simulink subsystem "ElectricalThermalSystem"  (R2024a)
settings: Solver=VariableStepAuto  StartTime=0.0  StopTime=10.0  RelTol=1e-3
undefined symbols (not defined in the file): EnvAirTemp, PlantThrEstCmpPwr, PlntThrAirBpt, PlntThrAirCond, PlntThrAirCp, PlntThrAirCpBpt, PlntThrAirPrand, PlntThrAirRho, PlntThrAirVisc, PlntThrBattDCFlwRatio, PlntThrBattJacLen, PlntThrChArea, PlntThrChDia, PlntThrCoolCond, PlntThrCoolCp, PlntThrCoolCpBpt, PlntThrCoolPrand, PlntThrCoolRho, PlntThrCoolVisc, PlntThrDCJacLen, PlntThrEMJacLen, PlntThrEstCOPLut, PlntThrEstDTLut, PlntThrHeaterMaxPwr, PlntThrPmpDisp, PlntThrPmpHeadP, PlntThrPmpMaxSpd, PlntThrPmpMechEff, PlntThrPmpVolEff, PlntThrRadAirArea, PlntThrRadAirDh, PlntThrRadFanAreaFlw, PlntThrRadFlwCoef, PlntThrRadGapHeight, PlntThrRadLength, PlntThrRadNTubes, PlntThrRadTubeDh, PlntThrRadTubeHeight, PlntThrRadWidth
libraries: autolibutils x45
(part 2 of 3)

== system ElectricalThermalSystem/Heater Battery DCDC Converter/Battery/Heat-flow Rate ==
  HTC : Inport
  JacHtArea : Inport  Port=2
  BattTemp : Inport  Port=3
  CoolBlkTemp : Inport  Port=4
  Product2 : Product  Inputs=3
  Subtract1 : Sum  Inputs=+-
  Qbatt : Outport
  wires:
  BattTemp/1 -> Subtract1/1
  Product2/1 -> Qbatt/1
  CoolBlkTemp/1 -> Subtract1/2
  JacHtArea/1 -> Product2/2
  Subtract1/1 -> Product2/3
  HTC/1 -> Product2/1

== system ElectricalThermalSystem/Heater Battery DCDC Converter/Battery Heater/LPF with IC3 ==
  u : Inport
  Cont LPF IC : autolibutils/Cont LPF IC  wc=wc  aMode=1  dataType=off
  Initial Condition : Constant  Value=InitCond  SampleTime=-1
  y : Outport
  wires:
  Cont LPF IC/1 -> y/1
  u/1 -> Cont LPF IC/1
  Initial Condition/1 -> Cont LPF IC/2

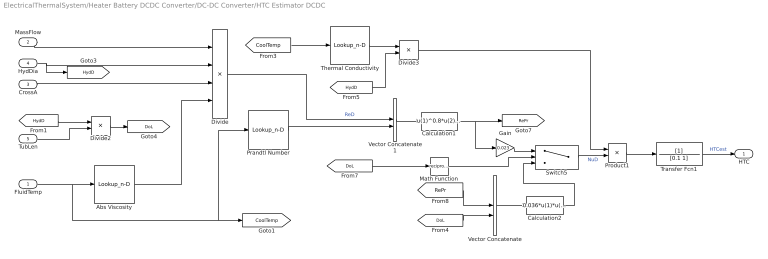
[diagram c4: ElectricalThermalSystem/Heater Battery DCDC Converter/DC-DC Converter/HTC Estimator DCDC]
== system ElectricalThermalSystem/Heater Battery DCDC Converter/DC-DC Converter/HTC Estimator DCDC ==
  FluidTemp : Inport
  MassFlow : Inport  Port=2
  CrossA : Inport  Port=3  OutMin=eps
  HydDia : Inport  Port=4
  TubLen : Inport  Port=5
  Abs Viscosity : Lookup_n-D  NumberOfTableDimensions=1  BreakpointsForDimension1=PlntThrCoolCpBpt  Table=PlntThrCoolVisc  ExtrapMethod=Clip  UseLastTableValue=on  InternalRulePriority=Speed  RndMeth=Simplest
  Calculation1 : Fcn  Expr=u(1)^0.8*u(2)^0.33
  Calculation2 : Fcn  Expr=0.036*u(1)*u(2)^0.055
  Divide : Product  Inputs=**//
  Divide2 : Product  Inputs=*/
  Divide3 : Product  Inputs=*/
  Gain : Gain  Gain=0.023
  Math Function : Math  Operator=reciprocal
  Prandtl Number : Lookup_n-D  NumberOfTableDimensions=1  BreakpointsForDimension1=PlntThrCoolCpBpt  Table=PlntThrCoolPrand  ExtrapMethod=Clip  UseLastTableValue=on  InternalRulePriority=Speed  RndMeth=Simplest
  Product1 : Product
  Switch5 : Switch  Threshold=400
  Thermal Conductivity : Lookup_n-D  NumberOfTableDimensions=1  BreakpointsForDimension1=PlntThrCoolCpBpt  Table=PlntThrCoolCond  ExtrapMethod=Clip  UseLastTableValue=on  InternalRulePriority=Speed  RndMeth=Simplest
  Transfer Fcn1 : TransferFcn  Denominator=[0.1 1]
  Vector Concatenate : Concatenate
  Vector Concatenate1 : Concatenate
  HTC : Outport
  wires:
  Product1/1 -> Transfer Fcn1/1
  Switch5/1 -> Product1/2  "NuD"
  Calculation2/1 -> Switch5/3
  Vector Concatenate/1 -> Calculation2/1
  [DoL] -> Vector Concatenate/2
  [RePr] -> Vector Concatenate/1
  Calculation1/1 -> Gain/1, [RePr]
  Gain/1 -> Switch5/1
  Divide3/1 -> Product1/1
  [HydD] -> Divide3/2
  Thermal Conductivity/1 -> Divide3/1
  Math Function/1 -> Switch5/2
  [DoL] -> Math Function/1
  Vector Concatenate1/1 -> Calculation1/1
  Prandtl Number/1 -> Vector Concatenate1/2
  Divide/1 -> Vector Concatenate1/1  "ReD"
  Abs Viscosity/1 -> Divide/4
  Divide2/1 -> [DoL]
  TubLen/1 -> Divide2/2
  [HydD] -> Divide2/1
  CrossA/1 -> Divide/3
  HydDia/1 -> Divide/2, [HydD]
  MassFlow/1 -> Divide/1
  [CoolTemp] -> Thermal Conductivity/1
  FluidTemp/1 -> Abs Viscosity/1, [CoolTemp], Prandtl Number/1
  Transfer Fcn1/1 -> HTC/1  "HTCest"

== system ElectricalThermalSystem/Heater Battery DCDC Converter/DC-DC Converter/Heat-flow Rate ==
  HTC : Inport
  PwrETemp : Inport  Port=2
  JacArea : Inport  Port=3
  CoolBlkTemp : Inport  Port=4
  Product1 : Product  Inputs=3
  Subtract : Sum  Inputs=+-
  Qpwre : Outport
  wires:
  HTC/1 -> Product1/1
  Product1/1 -> Qpwre/1
  CoolBlkTemp/1 -> Subtract/2
  PwrETemp/1 -> Subtract/1
  Subtract/1 -> Product1/3
  JacArea/1 -> Product1/2

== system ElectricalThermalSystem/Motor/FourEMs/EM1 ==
  CoolTempIn : Inport
  CoolMFlow : Inport  Port=2
  EMTemp : Inport  Port=3
  Constant : Constant  Value=JacHtArea  SampleTime=-1
  Constant1 : Constant  Value=JacDia
  Constant2 : Constant  Value=JacArea
  Constant3 : Constant  Value=JacLen
  HTC Estimator EM : Subsystem
  Temperature and Heat Flow : Subsystem
  Qem : Outport
  CoolTempOut : Outport  Port=2
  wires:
  Constant/1 -> Temperature and Heat Flow/5(JacArea)
  CoolTempIn/1 -> Temperature and Heat Flow/2(CoolTempIn)
  Temperature and Heat Flow/3(CoolTempOut) -> CoolTempOut/1
  Temperature and Heat Flow/2(Qem) -> Qem/1
  Constant2/1 -> HTC Estimator EM/3(CrossA)
  [BulkCoolTemp] -> HTC Estimator EM/1(FluidTemp)
  Constant3/1 -> HTC Estimator EM/5(TubLen)
  EMTemp/1 -> Temperature and Heat Flow/3(EMTemp)
  [CoolMFlw] -> Temperature and Heat Flow/4(CoolMflw)
  CoolMFlow/1 -> [CoolMFlw], HTC Estimator EM/2(MassFlow)
  HTC Estimator EM/1(HTC) -> Temperature and Heat Flow/1(HTC)
  Temperature and Heat Flow/1(BulkCoolTemp) -> [BulkCoolTemp]
  Constant1/1 -> HTC Estimator EM/4(HydDia)

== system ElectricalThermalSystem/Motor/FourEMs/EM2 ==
  CoolTempIn : Inport
  CoolMFlow : Inport  Port=2
  EMTemp : Inport  Port=3
  Constant : Constant  Value=JacHtArea  SampleTime=-1
  Constant1 : Constant  Value=JacDia
  Constant2 : Constant  Value=JacArea
  Constant3 : Constant  Value=JacLen
  HTC Estimator EM : Subsystem
  Temperature and Heat Flow : Subsystem
  Qem : Outport
  CoolTempOut : Outport  Port=2
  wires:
  Constant/1 -> Temperature and Heat Flow/5(JacArea)
  CoolTempIn/1 -> Temperature and Heat Flow/2(CoolTempIn)
  Temperature and Heat Flow/3(CoolTempOut) -> CoolTempOut/1
  Temperature and Heat Flow/2(Qem) -> Qem/1
  Constant2/1 -> HTC Estimator EM/3(CrossA)
  [BulkCoolTemp] -> HTC Estimator EM/1(FluidTemp)
  Constant3/1 -> HTC Estimator EM/5(TubLen)
  EMTemp/1 -> Temperature and Heat Flow/3(EMTemp)
  [CoolMFlw] -> Temperature and Heat Flow/4(CoolMflw)
  CoolMFlow/1 -> [CoolMFlw], HTC Estimator EM/2(MassFlow)
  HTC Estimator EM/1(HTC) -> Temperature and Heat Flow/1(HTC)
  Temperature and Heat Flow/1(BulkCoolTemp) -> [BulkCoolTemp]
  Constant1/1 -> HTC Estimator EM/4(HydDia)

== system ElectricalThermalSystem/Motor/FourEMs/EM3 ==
  CoolTempIn : Inport
  CoolMFlow : Inport  Port=2
  EMTemp : Inport  Port=3
  Constant : Constant  Value=JacHtArea  SampleTime=-1
  Constant1 : Constant  Value=JacDia
  Constant2 : Constant  Value=JacArea
  Constant3 : Constant  Value=JacLen
  HTC Estimator EM : Subsystem
  Temperature and Heat Flow : Subsystem
  Qem : Outport
  CoolTempOut : Outport  Port=2
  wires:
  Constant/1 -> Temperature and Heat Flow/5(JacArea)
  CoolTempIn/1 -> Temperature and Heat Flow/2(CoolTempIn)
  Temperature and Heat Flow/3(CoolTempOut) -> CoolTempOut/1
  Temperature and Heat Flow/2(Qem) -> Qem/1
  Constant2/1 -> HTC Estimator EM/3(CrossA)
  [BulkCoolTemp] -> HTC Estimator EM/1(FluidTemp)
  Constant3/1 -> HTC Estimator EM/5(TubLen)
  EMTemp/1 -> Temperature and Heat Flow/3(EMTemp)
  [CoolMFlw] -> Temperature and Heat Flow/4(CoolMflw)
  CoolMFlow/1 -> [CoolMFlw], HTC Estimator EM/2(MassFlow)
  HTC Estimator EM/1(HTC) -> Temperature and Heat Flow/1(HTC)
  Temperature and Heat Flow/1(BulkCoolTemp) -> [BulkCoolTemp]
  Constant1/1 -> HTC Estimator EM/4(HydDia)

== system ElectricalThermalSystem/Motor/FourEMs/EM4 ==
  CoolTempIn : Inport
  CoolMFlow : Inport  Port=2
  EMTemp : Inport  Port=3
  Constant : Constant  Value=JacHtArea  SampleTime=-1
  Constant1 : Constant  Value=JacDia
  Constant2 : Constant  Value=JacArea
  Constant3 : Constant  Value=JacLen
  HTC Estimator EM : Subsystem
  Temperature and Heat Flow : Subsystem
  Qem : Outport
  CoolTempOut : Outport  Port=2
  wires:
  Constant/1 -> Temperature and Heat Flow/5(JacArea)
  CoolTempIn/1 -> Temperature and Heat Flow/2(CoolTempIn)
  Temperature and Heat Flow/3(CoolTempOut) -> CoolTempOut/1
  Temperature and Heat Flow/2(Qem) -> Qem/1
  Constant2/1 -> HTC Estimator EM/3(CrossA)
  [BulkCoolTemp] -> HTC Estimator EM/1(FluidTemp)
  Constant3/1 -> HTC Estimator EM/5(TubLen)
  EMTemp/1 -> Temperature and Heat Flow/3(EMTemp)
  [CoolMFlw] -> Temperature and Heat Flow/4(CoolMflw)
  CoolMFlow/1 -> [CoolMFlw], HTC Estimator EM/2(MassFlow)
  HTC Estimator EM/1(HTC) -> Temperature and Heat Flow/1(HTC)
  Temperature and Heat Flow/1(BulkCoolTemp) -> [BulkCoolTemp]
  Constant1/1 -> HTC Estimator EM/4(HydDia)

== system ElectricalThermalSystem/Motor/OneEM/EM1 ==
  MassFlow : Inport
  CoolTempIn : Inport  Port=2
  EMTemp : Inport  Port=3
  Constant : Constant  Value=JacHtArea  SampleTime=-1
  Constant1 : Constant  Value=JacDia
  Constant2 : Constant  Value=JacArea
  Constant3 : Constant  Value=JacLen
  HTC Estimator EM : Subsystem
  Temperature and Heat Flow : Subsystem
  Qem : Outport
  CoolTempOut : Outport  Port=2
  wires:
  Constant/1 -> Temperature and Heat Flow/5(JacArea)
  CoolTempIn/1 -> Temperature and Heat Flow/2(CoolTempIn)
  Temperature and Heat Flow/3(CoolTempOut) -> CoolTempOut/1
  Temperature and Heat Flow/2(Qem) -> Qem/1
  Constant2/1 -> HTC Estimator EM/3(CrossA)
  [BulkCoolTemp] -> HTC Estimator EM/1(FluidTemp)
  Constant3/1 -> HTC Estimator EM/5(TubLen)
  EMTemp/1 -> Temperature and Heat Flow/3(EMTemp)
  [CoolMFlw] -> Temperature and Heat Flow/4(CoolMflw)
  MassFlow/1 -> [CoolMFlw], HTC Estimator EM/2(MassFlow)
  HTC Estimator EM/1(HTC) -> Temperature and Heat Flow/1(HTC)
  Temperature and Heat Flow/1(BulkCoolTemp) -> [BulkCoolTemp]
  Constant1/1 -> HTC Estimator EM/4(HydDia)

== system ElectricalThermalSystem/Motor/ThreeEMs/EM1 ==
  CoolTempIn : Inport
  CoolMFlow : Inport  Port=2
  EMTemp : Inport  Port=3
  Constant : Constant  Value=JacHtArea  SampleTime=-1
  Constant1 : Constant  Value=JacDia
  Constant2 : Constant  Value=JacArea
  Constant3 : Constant  Value=JacLen
  HTC Estimator EM : Subsystem
  Temperature and Heat Flow : Subsystem
  Qem : Outport
  CoolTempOut : Outport  Port=2
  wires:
  Constant/1 -> Temperature and Heat Flow/5(JacArea)
  CoolTempIn/1 -> Temperature and Heat Flow/2(CoolTempIn)
  Temperature and Heat Flow/3(CoolTempOut) -> CoolTempOut/1
  Temperature and Heat Flow/2(Qem) -> Qem/1
  Constant2/1 -> HTC Estimator EM/3(CrossA)
  [BulkCoolTemp] -> HTC Estimator EM/1(FluidTemp)
  Constant3/1 -> HTC Estimator EM/5(TubLen)
  EMTemp/1 -> Temperature and Heat Flow/3(EMTemp)
  [CoolMFlw] -> Temperature and Heat Flow/4(CoolMflw)
  CoolMFlow/1 -> [CoolMFlw], HTC Estimator EM/2(MassFlow)
  HTC Estimator EM/1(HTC) -> Temperature and Heat Flow/1(HTC)
  Temperature and Heat Flow/1(BulkCoolTemp) -> [BulkCoolTemp]
  Constant1/1 -> HTC Estimator EM/4(HydDia)

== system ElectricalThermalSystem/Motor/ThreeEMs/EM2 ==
  CoolTempIn : Inport
  CoolMFlow : Inport  Port=2
  EMTemp : Inport  Port=3
  Constant : Constant  Value=JacHtArea  SampleTime=-1
  Constant1 : Constant  Value=JacDia
  Constant2 : Constant  Value=JacArea
  Constant3 : Constant  Value=JacLen
  HTC Estimator EM : Subsystem
  Temperature and Heat Flow : Subsystem
  Qem : Outport
  CoolTempOut : Outport  Port=2
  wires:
  Constant/1 -> Temperature and Heat Flow/5(JacArea)
  CoolTempIn/1 -> Temperature and Heat Flow/2(CoolTempIn)
  Temperature and Heat Flow/3(CoolTempOut) -> CoolTempOut/1
  Temperature and Heat Flow/2(Qem) -> Qem/1
  Constant2/1 -> HTC Estimator EM/3(CrossA)
  [BulkCoolTemp] -> HTC Estimator EM/1(FluidTemp)
  Constant3/1 -> HTC Estimator EM/5(TubLen)
  EMTemp/1 -> Temperature and Heat Flow/3(EMTemp)
  [CoolMFlw] -> Temperature and Heat Flow/4(CoolMflw)
  CoolMFlow/1 -> [CoolMFlw], HTC Estimator EM/2(MassFlow)
  HTC Estimator EM/1(HTC) -> Temperature and Heat Flow/1(HTC)
  Temperature and Heat Flow/1(BulkCoolTemp) -> [BulkCoolTemp]
  Constant1/1 -> HTC Estimator EM/4(HydDia)

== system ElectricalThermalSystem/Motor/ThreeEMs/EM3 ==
  CoolTempIn : Inport
  CoolMFlow : Inport  Port=2
  EMTemp : Inport  Port=3
  Constant : Constant  Value=JacHtArea  SampleTime=-1
  Constant1 : Constant  Value=JacDia
  Constant2 : Constant  Value=JacArea
  Constant3 : Constant  Value=JacLen
  HTC Estimator EM : Subsystem
  Temperature and Heat Flow : Subsystem
  Qem : Outport
  CoolTempOut : Outport  Port=2
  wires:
  Constant/1 -> Temperature and Heat Flow/5(JacArea)
  CoolTempIn/1 -> Temperature and Heat Flow/2(CoolTempIn)
  Temperature and Heat Flow/3(CoolTempOut) -> CoolTempOut/1
  Temperature and Heat Flow/2(Qem) -> Qem/1
  Constant2/1 -> HTC Estimator EM/3(CrossA)
  [BulkCoolTemp] -> HTC Estimator EM/1(FluidTemp)
  Constant3/1 -> HTC Estimator EM/5(TubLen)
  EMTemp/1 -> Temperature and Heat Flow/3(EMTemp)
  [CoolMFlw] -> Temperature and Heat Flow/4(CoolMflw)
  CoolMFlow/1 -> [CoolMFlw], HTC Estimator EM/2(MassFlow)
  HTC Estimator EM/1(HTC) -> Temperature and Heat Flow/1(HTC)
  Temperature and Heat Flow/1(BulkCoolTemp) -> [BulkCoolTemp]
  Constant1/1 -> HTC Estimator EM/4(HydDia)

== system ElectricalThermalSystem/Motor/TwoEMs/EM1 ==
  CoolTempIn : Inport
  CoolMFlow : Inport  Port=2
  EMTemp : Inport  Port=3
  Constant : Constant  Value=JacHtArea  SampleTime=-1
  Constant1 : Constant  Value=JacDia
  Constant2 : Constant  Value=JacArea
  Constant3 : Constant  Value=JacLen
  HTC Estimator EM : Subsystem
  Temperature and Heat Flow : Subsystem
  Qem : Outport
  CoolTempOut : Outport  Port=2
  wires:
  Constant/1 -> Temperature and Heat Flow/5(JacArea)
  CoolTempIn/1 -> Temperature and Heat Flow/2(CoolTempIn)
  Temperature and Heat Flow/3(CoolTempOut) -> CoolTempOut/1
  Temperature and Heat Flow/2(Qem) -> Qem/1
  Constant2/1 -> HTC Estimator EM/3(CrossA)
  [BulkCoolTemp] -> HTC Estimator EM/1(FluidTemp)
  Constant3/1 -> HTC Estimator EM/5(TubLen)
  EMTemp/1 -> Temperature and Heat Flow/3(EMTemp)
  [CoolMFlw] -> Temperature and Heat Flow/4(CoolMflw)
  CoolMFlow/1 -> [CoolMFlw], HTC Estimator EM/2(MassFlow)
  HTC Estimator EM/1(HTC) -> Temperature and Heat Flow/1(HTC)
  Temperature and Heat Flow/1(BulkCoolTemp) -> [BulkCoolTemp]
  Constant1/1 -> HTC Estimator EM/4(HydDia)

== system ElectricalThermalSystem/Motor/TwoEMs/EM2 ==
  CoolTempIn : Inport
  CoolMFlow : Inport  Port=2
  EMTemp : Inport  Port=3
  Constant : Constant  Value=JacHtArea  SampleTime=-1
  Constant1 : Constant  Value=JacDia
  Constant2 : Constant  Value=JacArea
  Constant3 : Constant  Value=JacLen
  HTC Estimator EM : Subsystem
  Temperature and Heat Flow : Subsystem
  Qem : Outport
  CoolTempOut : Outport  Port=2
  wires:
  Constant/1 -> Temperature and Heat Flow/5(JacArea)
  CoolTempIn/1 -> Temperature and Heat Flow/2(CoolTempIn)
  Temperature and Heat Flow/3(CoolTempOut) -> CoolTempOut/1
  Temperature and Heat Flow/2(Qem) -> Qem/1
  Constant2/1 -> HTC Estimator EM/3(CrossA)
  [BulkCoolTemp] -> HTC Estimator EM/1(FluidTemp)
  Constant3/1 -> HTC Estimator EM/5(TubLen)
  EMTemp/1 -> Temperature and Heat Flow/3(EMTemp)
  [CoolMFlw] -> Temperature and Heat Flow/4(CoolMflw)
  CoolMFlow/1 -> [CoolMFlw], HTC Estimator EM/2(MassFlow)
  HTC Estimator EM/1(HTC) -> Temperature and Heat Flow/1(HTC)
  Temperature and Heat Flow/1(BulkCoolTemp) -> [BulkCoolTemp]
  Constant1/1 -> HTC Estimator EM/4(HydDia)

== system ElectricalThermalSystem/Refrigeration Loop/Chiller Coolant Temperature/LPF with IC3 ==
  u : Inport
  Cont LPF IC : autolibutils/Cont LPF IC  wc=wc  aMode=1  dataType=off
  Initial Condition : Constant  Value=InitCond  SampleTime=-1
  y : Outport
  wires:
  Cont LPF IC/1 -> y/1
  u/1 -> Cont LPF IC/1
  Initial Condition/1 -> Cont LPF IC/2

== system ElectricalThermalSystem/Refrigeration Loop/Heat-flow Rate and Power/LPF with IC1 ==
  u : Inport
  Cont LPF IC : autolibutils/Cont LPF IC  wc=wc  aMode=1  dataType=off
  Initial Condition : Constant  Value=InitCond  SampleTime=-1
  y : Outport
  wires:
  Cont LPF IC/1 -> y/1
  u/1 -> Cont LPF IC/1
  Initial Condition/1 -> Cont LPF IC/2

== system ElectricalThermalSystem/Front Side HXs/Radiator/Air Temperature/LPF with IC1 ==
  u : Inport
  Cont LPF IC : autolibutils/Cont LPF IC  wc=wc  aMode=1  dataType=off
  Initial Condition : Constant  Value=InitCond  SampleTime=-1
  y : Outport
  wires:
  Cont LPF IC/1 -> y/1
  u/1 -> Cont LPF IC/1
  Initial Condition/1 -> Cont LPF IC/2

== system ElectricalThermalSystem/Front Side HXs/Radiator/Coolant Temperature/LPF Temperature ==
  u : Inport
  Cont LPF IC : autolibutils/Cont LPF IC  wc=wc  aMode=1  dataType=off
  Initial Condition : Constant  Value=InitCond  SampleTime=-1
  y : Outport
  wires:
  Cont LPF IC/1 -> y/1
  u/1 -> Cont LPF IC/1
  Initial Condition/1 -> Cont LPF IC/2

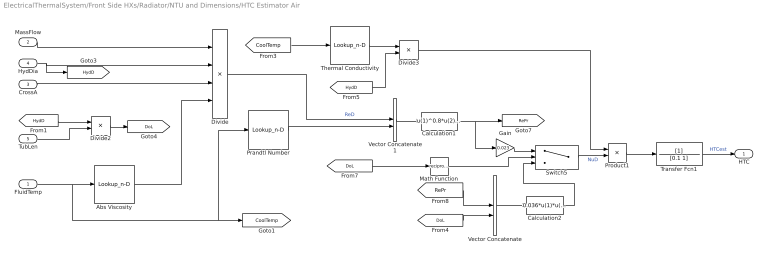
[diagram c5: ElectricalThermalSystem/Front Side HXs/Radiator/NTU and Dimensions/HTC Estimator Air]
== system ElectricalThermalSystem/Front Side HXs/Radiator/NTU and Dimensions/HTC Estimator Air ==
  FluidTemp : Inport
  MassFlow : Inport  Port=2
  CrossA : Inport  Port=3  OutMin=eps
  HydDia : Inport  Port=4
  TubLen : Inport  Port=5
  Abs Viscosity : Lookup_n-D  NumberOfTableDimensions=1  BreakpointsForDimension1=PlntThrAirCpBpt  Table=PlntThrAirVisc  ExtrapMethod=Clip  UseLastTableValue=on  InternalRulePriority=Speed  RndMeth=Simplest
  Calculation1 : Fcn  Expr=u(1)^0.8*u(2)^0.33
  Calculation2 : Fcn  Expr=0.036*u(1)*u(2)^0.055
  Divide : Product  Inputs=**//
  Divide2 : Product  Inputs=*/
  Divide3 : Product  Inputs=*/
  Gain : Gain  Gain=0.023
  Math Function : Math  Operator=reciprocal
  Prandtl Number : Lookup_n-D  NumberOfTableDimensions=1  BreakpointsForDimension1=PlntThrAirCpBpt  Table=PlntThrAirPrand  ExtrapMethod=Clip  UseLastTableValue=on  InternalRulePriority=Speed  RndMeth=Simplest
  Product1 : Product
  Switch5 : Switch  Threshold=400
  Thermal Conductivity : Lookup_n-D  NumberOfTableDimensions=1  BreakpointsForDimension1=PlntThrAirCpBpt  Table=PlntThrAirCond  ExtrapMethod=Clip  UseLastTableValue=on  InternalRulePriority=Speed  RndMeth=Simplest
  Transfer Fcn1 : TransferFcn  Denominator=[0.1 1]
  Vector Concatenate : Concatenate
  Vector Concatenate1 : Concatenate
  HTC : Outport
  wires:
  MassFlow/1 -> Divide/1
  Product1/1 -> Transfer Fcn1/1
  Switch5/1 -> Product1/2  "NuD"
  Calculation2/1 -> Switch5/3
  Vector Concatenate/1 -> Calculation2/1
  [DoL] -> Vector Concatenate/2
  [RePr] -> Vector Concatenate/1
  Calculation1/1 -> Gain/1, [RePr]
  Gain/1 -> Switch5/1
  Divide3/1 -> Product1/1
  [HydD] -> Divide3/2
  Thermal Conductivity/1 -> Divide3/1
  Math Function/1 -> Switch5/2
  [DoL] -> Math Function/1
  Vector Concatenate1/1 -> Calculation1/1
  Prandtl Number/1 -> Vector Concatenate1/2
  Divide/1 -> Vector Concatenate1/1  "ReD"
  Abs Viscosity/1 -> Divide/4
  Divide2/1 -> [DoL]
  TubLen/1 -> Divide2/2
  [HydD] -> Divide2/1
  CrossA/1 -> Divide/3
  HydDia/1 -> Divide/2, [HydD]
  [CoolTemp] -> Thermal Conductivity/1
  FluidTemp/1 -> Abs Viscosity/1, [CoolTemp], Prandtl Number/1
  Transfer Fcn1/1 -> HTC/1  "HTCest"

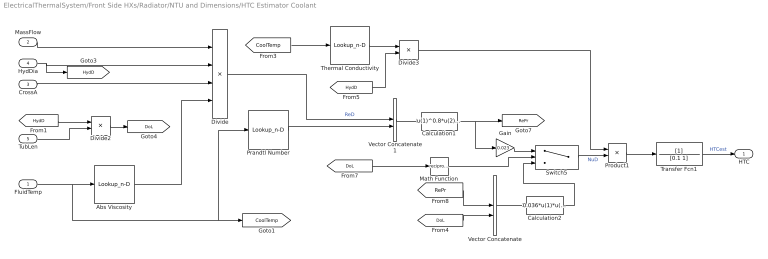
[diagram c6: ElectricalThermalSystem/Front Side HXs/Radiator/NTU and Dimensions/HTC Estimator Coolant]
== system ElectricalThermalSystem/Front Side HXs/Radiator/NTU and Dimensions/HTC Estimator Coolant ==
  FluidTemp : Inport
  MassFlow : Inport  Port=2
  CrossA : Inport  Port=3  OutMin=eps
  HydDia : Inport  Port=4
  TubLen : Inport  Port=5
  Abs Viscosity : Lookup_n-D  NumberOfTableDimensions=1  BreakpointsForDimension1=PlntThrCoolCpBpt  Table=PlntThrCoolVisc  ExtrapMethod=Clip  UseLastTableValue=on  InternalRulePriority=Speed  RndMeth=Simplest
  Calculation1 : Fcn  Expr=u(1)^0.8*u(2)^0.33
  Calculation2 : Fcn  Expr=0.036*u(1)*u(2)^0.055
  Divide : Product  Inputs=**//
  Divide2 : Product  Inputs=*/
  Divide3 : Product  Inputs=*/
  Gain : Gain  Gain=0.023
  Math Function : Math  Operator=reciprocal
  Prandtl Number : Lookup_n-D  NumberOfTableDimensions=1  BreakpointsForDimension1=PlntThrCoolCpBpt  Table=PlntThrCoolPrand  ExtrapMethod=Clip  UseLastTableValue=on  InternalRulePriority=Speed  RndMeth=Simplest
  Product1 : Product
  Switch5 : Switch  Threshold=400
  Thermal Conductivity : Lookup_n-D  NumberOfTableDimensions=1  BreakpointsForDimension1=PlntThrCoolCpBpt  Table=PlntThrCoolCond  ExtrapMethod=Clip  UseLastTableValue=on  InternalRulePriority=Speed  RndMeth=Simplest
  Transfer Fcn1 : TransferFcn  Denominator=[0.1 1]
  Vector Concatenate : Concatenate
  Vector Concatenate1 : Concatenate
  HTC : Outport
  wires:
  MassFlow/1 -> Divide/1
  Product1/1 -> Transfer Fcn1/1
  Switch5/1 -> Product1/2  "NuD"
  Calculation2/1 -> Switch5/3
  Vector Concatenate/1 -> Calculation2/1
  [DoL] -> Vector Concatenate/2
  [RePr] -> Vector Concatenate/1
  Calculation1/1 -> Gain/1, [RePr]
  Gain/1 -> Switch5/1
  Divide3/1 -> Product1/1
  [HydD] -> Divide3/2
  Thermal Conductivity/1 -> Divide3/1
  Math Function/1 -> Switch5/2
  [DoL] -> Math Function/1
  Vector Concatenate1/1 -> Calculation1/1
  Prandtl Number/1 -> Vector Concatenate1/2
  Divide/1 -> Vector Concatenate1/1  "ReD"
  Abs Viscosity/1 -> Divide/4
  Divide2/1 -> [DoL]
  TubLen/1 -> Divide2/2
  [HydD] -> Divide2/1
  CrossA/1 -> Divide/3
  HydDia/1 -> Divide/2, [HydD]
  [CoolTemp] -> Thermal Conductivity/1
  FluidTemp/1 -> Abs Viscosity/1, [CoolTemp], Prandtl Number/1
  Transfer Fcn1/1 -> HTC/1  "HTCest"

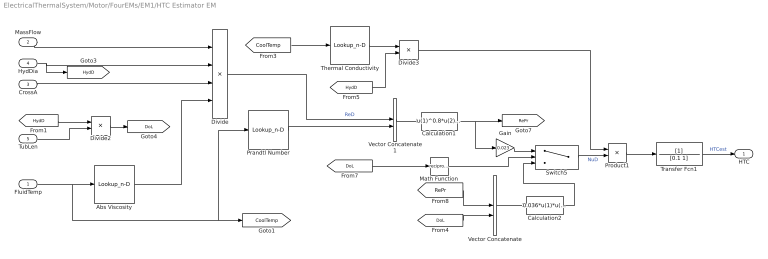
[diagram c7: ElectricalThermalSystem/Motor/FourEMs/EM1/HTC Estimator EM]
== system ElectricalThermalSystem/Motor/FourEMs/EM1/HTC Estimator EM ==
  FluidTemp : Inport
  MassFlow : Inport  Port=2
  CrossA : Inport  Port=3  OutMin=eps
  HydDia : Inport  Port=4
  TubLen : Inport  Port=5
  Abs Viscosity : Lookup_n-D  NumberOfTableDimensions=1  BreakpointsForDimension1=PlntThrCoolCpBpt  Table=PlntThrCoolVisc  ExtrapMethod=Clip  UseLastTableValue=on  InternalRulePriority=Speed  RndMeth=Simplest
  Calculation1 : Fcn  Expr=u(1)^0.8*u(2)^0.33
  Calculation2 : Fcn  Expr=0.036*u(1)*u(2)^0.055
  Divide : Product  Inputs=**//
  Divide2 : Product  Inputs=*/
  Divide3 : Product  Inputs=*/
  Gain : Gain  Gain=0.023
  Math Function : Math  Operator=reciprocal
  Prandtl Number : Lookup_n-D  NumberOfTableDimensions=1  BreakpointsForDimension1=PlntThrCoolCpBpt  Table=PlntThrCoolPrand  ExtrapMethod=Clip  UseLastTableValue=on  InternalRulePriority=Speed  RndMeth=Simplest
  Product1 : Product
  Switch5 : Switch  Threshold=400
  Thermal Conductivity : Lookup_n-D  NumberOfTableDimensions=1  BreakpointsForDimension1=PlntThrCoolCpBpt  Table=PlntThrCoolCond  ExtrapMethod=Clip  UseLastTableValue=on  InternalRulePriority=Speed  RndMeth=Simplest
  Transfer Fcn1 : TransferFcn  Denominator=[0.1 1]
  Vector Concatenate : Concatenate
  Vector Concatenate1 : Concatenate
  HTC : Outport
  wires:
  Transfer Fcn1/1 -> HTC/1  "HTCest"
  FluidTemp/1 -> Prandtl Number/1, [CoolTemp], Abs Viscosity/1
  [CoolTemp] -> Thermal Conductivity/1
  MassFlow/1 -> Divide/1
  HydDia/1 -> [HydD], Divide/2
  CrossA/1 -> Divide/3
  [HydD] -> Divide2/1
  TubLen/1 -> Divide2/2
  Divide2/1 -> [DoL]
  Abs Viscosity/1 -> Divide/4
  Divide/1 -> Vector Concatenate1/1  "ReD"
  Prandtl Number/1 -> Vector Concatenate1/2
  Vector Concatenate1/1 -> Calculation1/1
  [DoL] -> Math Function/1
  Math Function/1 -> Switch5/2
  Thermal Conductivity/1 -> Divide3/1
  [HydD] -> Divide3/2
  Divide3/1 -> Product1/1
  Gain/1 -> Switch5/1
  Calculation1/1 -> [RePr], Gain/1
  [RePr] -> Vector Concatenate/1
  [DoL] -> Vector Concatenate/2
  Vector Concatenate/1 -> Calculation2/1
  Calculation2/1 -> Switch5/3
  Switch5/1 -> Product1/2  "NuD"
  Product1/1 -> Transfer Fcn1/1

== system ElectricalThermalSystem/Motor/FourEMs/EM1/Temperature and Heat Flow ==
  HTC : Inport
  CoolTempIn : Inport  Port=2
  EMTemp : Inport  Port=3
  CoolMflw : Inport  Port=4
  JacArea : Inport  Port=5
  Divide2 : Product  Inputs=*/
  Gain4 : Gain  Gain=0.5
  LPF with IC1 : Subsystem  mask{wc=10, InitCond=EnvAirTemp, dataType=off}
      mask prompts: wc "Cutoff frequency, wc [rad/s]"; InitCond "Initial condition, InitCond [same as u]"; dataType "Enforce same input data type"
  Minus3 : Sum
  Minus4 : Sum
  Product1 : Product  Inputs=3
  Product2 : Product
  Selector : Selector  InputPortWidth=PlntEMNum  IndexOptions=Index vector (dialog)  Indices=1  OutputSizes=1
  Specific Heat 2 : Lookup_n-D  NumberOfTableDimensions=1  BreakpointsForDimension1=PlntThrCoolCpBpt  Table=PlntThrCoolCp  ExtrapMethod=Clip  UseLastTableValue=on  InternalRulePriority=Speed  RndMeth=Simplest
  Subtract : Sum  Inputs=+-
  div0protect - abs poly4 : autolibutils/div0protect - abs poly  thresh=.001  aMode=1
  BulkCoolTemp : Outport
  Qem : Outport  Port=2
  CoolTempOut : Outport  Port=3
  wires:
  LPF with IC1/1(y) -> BulkCoolTemp/1, [BulkCoolTemp]
  EMTemp/1 -> Selector/1
  HTC/1 -> Product1/1
  Product2/1 -> div0protect - abs poly4/1
  Minus4/1 -> Gain4/1
  Gain4/1 -> LPF with IC1/1(u)
  Minus3/1 -> Minus4/2, CoolTempOut/1
  Product1/1 -> Divide2/1, Qem/1  "Qem"
  JacArea/1 -> Product1/2
  div0protect - abs poly4/1 -> Divide2/2
  Specific Heat 2/1 -> Product2/2
  [BulkCoolTemp] -> Specific Heat 2/1, Subtract/2
  Subtract/1 -> Product1/3
  Selector/1 -> Subtract/1
  Divide2/1 -> Minus3/2
  CoolMflw/1 -> Product2/1
  CoolTempIn/1 -> Minus4/1, Minus3/1

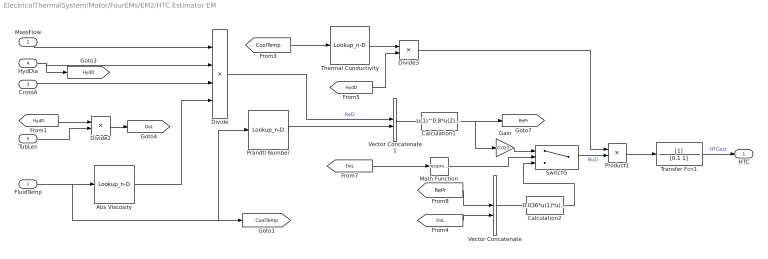
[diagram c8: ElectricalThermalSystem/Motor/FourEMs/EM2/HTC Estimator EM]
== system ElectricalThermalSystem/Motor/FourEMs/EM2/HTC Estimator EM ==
  FluidTemp : Inport
  MassFlow : Inport  Port=2
  CrossA : Inport  Port=3  OutMin=eps
  HydDia : Inport  Port=4
  TubLen : Inport  Port=5
  Abs Viscosity : Lookup_n-D  NumberOfTableDimensions=1  BreakpointsForDimension1=PlntThrCoolCpBpt  Table=PlntThrCoolVisc  ExtrapMethod=Clip  UseLastTableValue=on  InternalRulePriority=Speed  RndMeth=Simplest
  Calculation1 : Fcn  Expr=u(1)^0.8*u(2)^0.33
  Calculation2 : Fcn  Expr=0.036*u(1)*u(2)^0.055
  Divide : Product  Inputs=**//
  Divide2 : Product  Inputs=*/
  Divide3 : Product  Inputs=*/
  Gain : Gain  Gain=0.023
  Math Function : Math  Operator=reciprocal
  Prandtl Number : Lookup_n-D  NumberOfTableDimensions=1  BreakpointsForDimension1=PlntThrCoolCpBpt  Table=PlntThrCoolPrand  ExtrapMethod=Clip  UseLastTableValue=on  InternalRulePriority=Speed  RndMeth=Simplest
  Product1 : Product
  Switch5 : Switch  Threshold=400
  Thermal Conductivity : Lookup_n-D  NumberOfTableDimensions=1  BreakpointsForDimension1=PlntThrCoolCpBpt  Table=PlntThrCoolCond  ExtrapMethod=Clip  UseLastTableValue=on  InternalRulePriority=Speed  RndMeth=Simplest
  Transfer Fcn1 : TransferFcn  Denominator=[0.1 1]
  Vector Concatenate : Concatenate
  Vector Concatenate1 : Concatenate
  HTC : Outport
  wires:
  Transfer Fcn1/1 -> HTC/1  "HTCest"
  FluidTemp/1 -> Prandtl Number/1, [CoolTemp], Abs Viscosity/1
  [CoolTemp] -> Thermal Conductivity/1
  MassFlow/1 -> Divide/1
  HydDia/1 -> [HydD], Divide/2
  CrossA/1 -> Divide/3
  [HydD] -> Divide2/1
  TubLen/1 -> Divide2/2
  Divide2/1 -> [DoL]
  Abs Viscosity/1 -> Divide/4
  Divide/1 -> Vector Concatenate1/1  "ReD"
  Prandtl Number/1 -> Vector Concatenate1/2
  Vector Concatenate1/1 -> Calculation1/1
  [DoL] -> Math Function/1
  Math Function/1 -> Switch5/2
  Thermal Conductivity/1 -> Divide3/1
  [HydD] -> Divide3/2
  Divide3/1 -> Product1/1
  Gain/1 -> Switch5/1
  Calculation1/1 -> [RePr], Gain/1
  [RePr] -> Vector Concatenate/1
  [DoL] -> Vector Concatenate/2
  Vector Concatenate/1 -> Calculation2/1
  Calculation2/1 -> Switch5/3
  Switch5/1 -> Product1/2  "NuD"
  Product1/1 -> Transfer Fcn1/1

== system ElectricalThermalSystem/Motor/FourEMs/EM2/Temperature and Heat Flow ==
  HTC : Inport
  CoolTempIn : Inport  Port=2
  EMTemp : Inport  Port=3
  CoolMflw : Inport  Port=4
  JacArea : Inport  Port=5
  Divide2 : Product  Inputs=*/
  Gain4 : Gain  Gain=0.5
  LPF with IC1 : Subsystem  mask{wc=10, InitCond=EnvAirTemp, dataType=off}
      mask prompts: wc "Cutoff frequency, wc [rad/s]"; InitCond "Initial condition, InitCond [same as u]"; dataType "Enforce same input data type"
  Minus3 : Sum
  Minus4 : Sum
  Product1 : Product  Inputs=3
  Product2 : Product
  Selector : Selector  InputPortWidth=PlntEMNum  IndexOptions=Index vector (dialog)  Indices=2  OutputSizes=1
  Specific Heat 2 : Lookup_n-D  NumberOfTableDimensions=1  BreakpointsForDimension1=PlntThrCoolCpBpt  Table=PlntThrCoolCp  ExtrapMethod=Clip  UseLastTableValue=on  InternalRulePriority=Speed  RndMeth=Simplest
  Subtract : Sum  Inputs=+-
  div0protect - abs poly4 : autolibutils/div0protect - abs poly  thresh=.001  aMode=1
  BulkCoolTemp : Outport
  Qem : Outport  Port=2
  CoolTempOut : Outport  Port=3
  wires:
  LPF with IC1/1(y) -> BulkCoolTemp/1, [BulkCoolTemp]
  EMTemp/1 -> Selector/1
  HTC/1 -> Product1/1
  Product2/1 -> div0protect - abs poly4/1
  Minus4/1 -> Gain4/1
  Gain4/1 -> LPF with IC1/1(u)
  Minus3/1 -> Minus4/2, CoolTempOut/1
  Product1/1 -> Divide2/1, Qem/1  "Qem"
  JacArea/1 -> Product1/2
  div0protect - abs poly4/1 -> Divide2/2
  Specific Heat 2/1 -> Product2/2
  [BulkCoolTemp] -> Specific Heat 2/1, Subtract/2
  Subtract/1 -> Product1/3
  Selector/1 -> Subtract/1
  Divide2/1 -> Minus3/2
  CoolMflw/1 -> Product2/1
  CoolTempIn/1 -> Minus4/1, Minus3/1

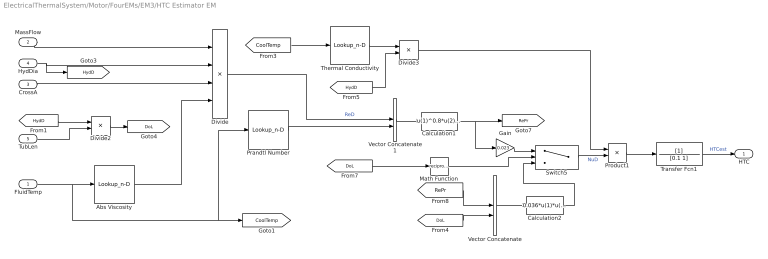
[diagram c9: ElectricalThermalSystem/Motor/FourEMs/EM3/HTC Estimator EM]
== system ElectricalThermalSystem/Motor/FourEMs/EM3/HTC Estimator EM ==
  FluidTemp : Inport
  MassFlow : Inport  Port=2
  CrossA : Inport  Port=3  OutMin=eps
  HydDia : Inport  Port=4
  TubLen : Inport  Port=5
  Abs Viscosity : Lookup_n-D  NumberOfTableDimensions=1  BreakpointsForDimension1=PlntThrCoolCpBpt  Table=PlntThrCoolVisc  ExtrapMethod=Clip  UseLastTableValue=on  InternalRulePriority=Speed  RndMeth=Simplest
  Calculation1 : Fcn  Expr=u(1)^0.8*u(2)^0.33
  Calculation2 : Fcn  Expr=0.036*u(1)*u(2)^0.055
  Divide : Product  Inputs=**//
  Divide2 : Product  Inputs=*/
  Divide3 : Product  Inputs=*/
  Gain : Gain  Gain=0.023
  Math Function : Math  Operator=reciprocal
  Prandtl Number : Lookup_n-D  NumberOfTableDimensions=1  BreakpointsForDimension1=PlntThrCoolCpBpt  Table=PlntThrCoolPrand  ExtrapMethod=Clip  UseLastTableValue=on  InternalRulePriority=Speed  RndMeth=Simplest
  Product1 : Product
  Switch5 : Switch  Threshold=400
  Thermal Conductivity : Lookup_n-D  NumberOfTableDimensions=1  BreakpointsForDimension1=PlntThrCoolCpBpt  Table=PlntThrCoolCond  ExtrapMethod=Clip  UseLastTableValue=on  InternalRulePriority=Speed  RndMeth=Simplest
  Transfer Fcn1 : TransferFcn  Denominator=[0.1 1]
  Vector Concatenate : Concatenate
  Vector Concatenate1 : Concatenate
  HTC : Outport
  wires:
  Transfer Fcn1/1 -> HTC/1  "HTCest"
  FluidTemp/1 -> Prandtl Number/1, [CoolTemp], Abs Viscosity/1
  [CoolTemp] -> Thermal Conductivity/1
  MassFlow/1 -> Divide/1
  HydDia/1 -> [HydD], Divide/2
  CrossA/1 -> Divide/3
  [HydD] -> Divide2/1
  TubLen/1 -> Divide2/2
  Divide2/1 -> [DoL]
  Abs Viscosity/1 -> Divide/4
  Divide/1 -> Vector Concatenate1/1  "ReD"
  Prandtl Number/1 -> Vector Concatenate1/2
  Vector Concatenate1/1 -> Calculation1/1
  [DoL] -> Math Function/1
  Math Function/1 -> Switch5/2
  Thermal Conductivity/1 -> Divide3/1
  [HydD] -> Divide3/2
  Divide3/1 -> Product1/1
  Gain/1 -> Switch5/1
  Calculation1/1 -> [RePr], Gain/1
  [RePr] -> Vector Concatenate/1
  [DoL] -> Vector Concatenate/2
  Vector Concatenate/1 -> Calculation2/1
  Calculation2/1 -> Switch5/3
  Switch5/1 -> Product1/2  "NuD"
  Product1/1 -> Transfer Fcn1/1

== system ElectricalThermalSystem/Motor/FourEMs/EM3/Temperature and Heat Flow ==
  HTC : Inport
  CoolTempIn : Inport  Port=2
  EMTemp : Inport  Port=3
  CoolMflw : Inport  Port=4
  JacArea : Inport  Port=5
  Divide2 : Product  Inputs=*/
  Gain4 : Gain  Gain=0.5
  LPF with IC1 : Subsystem  mask{wc=10, InitCond=EnvAirTemp, dataType=off}
      mask prompts: wc "Cutoff frequency, wc [rad/s]"; InitCond "Initial condition, InitCond [same as u]"; dataType "Enforce same input data type"
  Minus3 : Sum
  Minus4 : Sum
  Product1 : Product  Inputs=3
  Product2 : Product
  Selector : Selector  InputPortWidth=PlntEMNum  IndexOptions=Index vector (dialog)  Indices=3  OutputSizes=1
  Specific Heat 2 : Lookup_n-D  NumberOfTableDimensions=1  BreakpointsForDimension1=PlntThrCoolCpBpt  Table=PlntThrCoolCp  ExtrapMethod=Clip  UseLastTableValue=on  InternalRulePriority=Speed  RndMeth=Simplest
  Subtract : Sum  Inputs=+-
  div0protect - abs poly4 : autolibutils/div0protect - abs poly  thresh=.001  aMode=1
  BulkCoolTemp : Outport
  Qem : Outport  Port=2
  CoolTempOut : Outport  Port=3
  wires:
  LPF with IC1/1(y) -> BulkCoolTemp/1, [BulkCoolTemp]
  EMTemp/1 -> Selector/1
  HTC/1 -> Product1/1
  Product2/1 -> div0protect - abs poly4/1
  Minus4/1 -> Gain4/1
  Gain4/1 -> LPF with IC1/1(u)
  Minus3/1 -> Minus4/2, CoolTempOut/1
  Product1/1 -> Divide2/1, Qem/1  "Qem"
  JacArea/1 -> Product1/2
  div0protect - abs poly4/1 -> Divide2/2
  Specific Heat 2/1 -> Product2/2
  [BulkCoolTemp] -> Specific Heat 2/1, Subtract/2
  Subtract/1 -> Product1/3
  Selector/1 -> Subtract/1
  Divide2/1 -> Minus3/2
  CoolMflw/1 -> Product2/1
  CoolTempIn/1 -> Minus4/1, Minus3/1

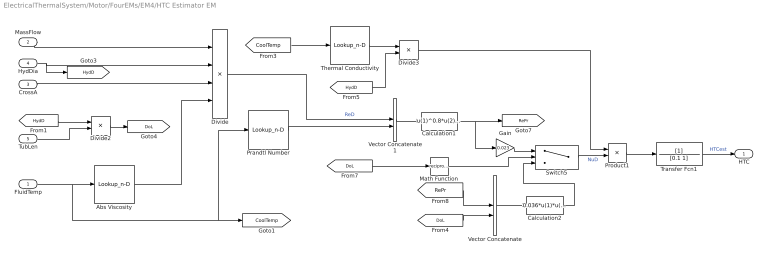
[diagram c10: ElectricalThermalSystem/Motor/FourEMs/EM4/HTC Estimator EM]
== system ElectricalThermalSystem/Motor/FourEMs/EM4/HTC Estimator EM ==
  FluidTemp : Inport
  MassFlow : Inport  Port=2
  CrossA : Inport  Port=3  OutMin=eps
  HydDia : Inport  Port=4
  TubLen : Inport  Port=5
  Abs Viscosity : Lookup_n-D  NumberOfTableDimensions=1  BreakpointsForDimension1=PlntThrCoolCpBpt  Table=PlntThrCoolVisc  ExtrapMethod=Clip  UseLastTableValue=on  InternalRulePriority=Speed  RndMeth=Simplest
  Calculation1 : Fcn  Expr=u(1)^0.8*u(2)^0.33
  Calculation2 : Fcn  Expr=0.036*u(1)*u(2)^0.055
  Divide : Product  Inputs=**//
  Divide2 : Product  Inputs=*/
  Divide3 : Product  Inputs=*/
  Gain : Gain  Gain=0.023
  Math Function : Math  Operator=reciprocal
  Prandtl Number : Lookup_n-D  NumberOfTableDimensions=1  BreakpointsForDimension1=PlntThrCoolCpBpt  Table=PlntThrCoolPrand  ExtrapMethod=Clip  UseLastTableValue=on  InternalRulePriority=Speed  RndMeth=Simplest
  Product1 : Product
  Switch5 : Switch  Threshold=400
  Thermal Conductivity : Lookup_n-D  NumberOfTableDimensions=1  BreakpointsForDimension1=PlntThrCoolCpBpt  Table=PlntThrCoolCond  ExtrapMethod=Clip  UseLastTableValue=on  InternalRulePriority=Speed  RndMeth=Simplest
  Transfer Fcn1 : TransferFcn  Denominator=[0.1 1]
  Vector Concatenate : Concatenate
  Vector Concatenate1 : Concatenate
  HTC : Outport
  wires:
  Transfer Fcn1/1 -> HTC/1  "HTCest"
  FluidTemp/1 -> Prandtl Number/1, [CoolTemp], Abs Viscosity/1
  [CoolTemp] -> Thermal Conductivity/1
  MassFlow/1 -> Divide/1
  HydDia/1 -> [HydD], Divide/2
  CrossA/1 -> Divide/3
  [HydD] -> Divide2/1
  TubLen/1 -> Divide2/2
  Divide2/1 -> [DoL]
  Abs Viscosity/1 -> Divide/4
  Divide/1 -> Vector Concatenate1/1  "ReD"
  Prandtl Number/1 -> Vector Concatenate1/2
  Vector Concatenate1/1 -> Calculation1/1
  [DoL] -> Math Function/1
  Math Function/1 -> Switch5/2
  Thermal Conductivity/1 -> Divide3/1
  [HydD] -> Divide3/2
  Divide3/1 -> Product1/1
  Gain/1 -> Switch5/1
  Calculation1/1 -> [RePr], Gain/1
  [RePr] -> Vector Concatenate/1
  [DoL] -> Vector Concatenate/2
  Vector Concatenate/1 -> Calculation2/1
  Calculation2/1 -> Switch5/3
  Switch5/1 -> Product1/2  "NuD"
  Product1/1 -> Transfer Fcn1/1

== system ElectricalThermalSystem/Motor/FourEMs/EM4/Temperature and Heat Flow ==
  HTC : Inport
  CoolTempIn : Inport  Port=2
  EMTemp : Inport  Port=3
  CoolMflw : Inport  Port=4
  JacArea : Inport  Port=5
  Divide2 : Product  Inputs=*/
  Gain4 : Gain  Gain=0.5
  LPF with IC1 : Subsystem  mask{wc=10, InitCond=EnvAirTemp, dataType=off}
      mask prompts: wc "Cutoff frequency, wc [rad/s]"; InitCond "Initial condition, InitCond [same as u]"; dataType "Enforce same input data type"
  Minus3 : Sum
  Minus4 : Sum
  Product1 : Product  Inputs=3
  Product2 : Product
  Selector : Selector  InputPortWidth=PlntEMNum  IndexOptions=Index vector (dialog)  Indices=4  OutputSizes=1
  Specific Heat 2 : Lookup_n-D  NumberOfTableDimensions=1  BreakpointsForDimension1=PlntThrCoolCpBpt  Table=PlntThrCoolCp  ExtrapMethod=Clip  UseLastTableValue=on  InternalRulePriority=Speed  RndMeth=Simplest
  Subtract : Sum  Inputs=+-
  div0protect - abs poly4 : autolibutils/div0protect - abs poly  thresh=.001  aMode=1
  BulkCoolTemp : Outport
  Qem : Outport  Port=2
  CoolTempOut : Outport  Port=3
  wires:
  LPF with IC1/1(y) -> BulkCoolTemp/1, [BulkCoolTemp]
  EMTemp/1 -> Selector/1
  HTC/1 -> Product1/1
  Product2/1 -> div0protect - abs poly4/1
  Minus4/1 -> Gain4/1
  Gain4/1 -> LPF with IC1/1(u)
  Minus3/1 -> Minus4/2, CoolTempOut/1
  Product1/1 -> Divide2/1, Qem/1  "Qem"
  JacArea/1 -> Product1/2
  div0protect - abs poly4/1 -> Divide2/2
  Specific Heat 2/1 -> Product2/2
  [BulkCoolTemp] -> Specific Heat 2/1, Subtract/2
  Subtract/1 -> Product1/3
  Selector/1 -> Subtract/1
  Divide2/1 -> Minus3/2
  CoolMflw/1 -> Product2/1
  CoolTempIn/1 -> Minus4/1, Minus3/1

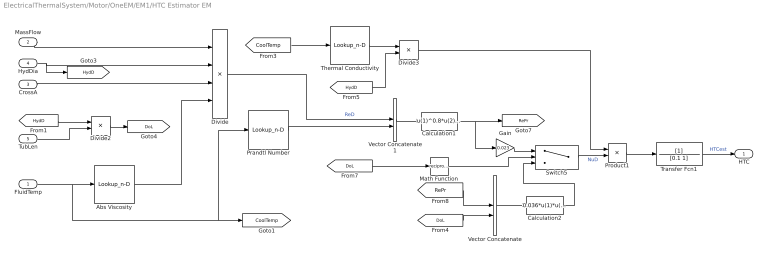
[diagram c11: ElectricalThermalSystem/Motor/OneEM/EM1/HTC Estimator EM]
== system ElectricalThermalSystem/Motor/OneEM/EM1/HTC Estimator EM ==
  FluidTemp : Inport
  MassFlow : Inport  Port=2
  CrossA : Inport  Port=3  OutMin=eps
  HydDia : Inport  Port=4
  TubLen : Inport  Port=5
  Abs Viscosity : Lookup_n-D  NumberOfTableDimensions=1  BreakpointsForDimension1=PlntThrCoolCpBpt  Table=PlntThrCoolVisc  ExtrapMethod=Clip  UseLastTableValue=on  InternalRulePriority=Speed  RndMeth=Simplest
  Calculation1 : Fcn  Expr=u(1)^0.8*u(2)^0.33
  Calculation2 : Fcn  Expr=0.036*u(1)*u(2)^0.055
  Divide : Product  Inputs=**//
  Divide2 : Product  Inputs=*/
  Divide3 : Product  Inputs=*/
  Gain : Gain  Gain=0.023
  Math Function : Math  Operator=reciprocal
  Prandtl Number : Lookup_n-D  NumberOfTableDimensions=1  BreakpointsForDimension1=PlntThrCoolCpBpt  Table=PlntThrCoolPrand  ExtrapMethod=Clip  UseLastTableValue=on  InternalRulePriority=Speed  RndMeth=Simplest
  Product1 : Product
  Switch5 : Switch  Threshold=400
  Thermal Conductivity : Lookup_n-D  NumberOfTableDimensions=1  BreakpointsForDimension1=PlntThrCoolCpBpt  Table=PlntThrCoolCond  ExtrapMethod=Clip  UseLastTableValue=on  InternalRulePriority=Speed  RndMeth=Simplest
  Transfer Fcn1 : TransferFcn  Denominator=[0.1 1]
  Vector Concatenate : Concatenate
  Vector Concatenate1 : Concatenate
  HTC : Outport
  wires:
  Transfer Fcn1/1 -> HTC/1  "HTCest"
  FluidTemp/1 -> Prandtl Number/1, [CoolTemp], Abs Viscosity/1
  [CoolTemp] -> Thermal Conductivity/1
  MassFlow/1 -> Divide/1
  HydDia/1 -> [HydD], Divide/2
  CrossA/1 -> Divide/3
  [HydD] -> Divide2/1
  TubLen/1 -> Divide2/2
  Divide2/1 -> [DoL]
  Abs Viscosity/1 -> Divide/4
  Divide/1 -> Vector Concatenate1/1  "ReD"
  Prandtl Number/1 -> Vector Concatenate1/2
  Vector Concatenate1/1 -> Calculation1/1
  [DoL] -> Math Function/1
  Math Function/1 -> Switch5/2
  Thermal Conductivity/1 -> Divide3/1
  [HydD] -> Divide3/2
  Divide3/1 -> Product1/1
  Gain/1 -> Switch5/1
  Calculation1/1 -> [RePr], Gain/1
  [RePr] -> Vector Concatenate/1
  [DoL] -> Vector Concatenate/2
  Vector Concatenate/1 -> Calculation2/1
  Calculation2/1 -> Switch5/3
  Switch5/1 -> Product1/2  "NuD"
  Product1/1 -> Transfer Fcn1/1

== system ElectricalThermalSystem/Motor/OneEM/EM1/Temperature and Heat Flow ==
  HTC : Inport
  CoolTempIn : Inport  Port=2
  EMTemp : Inport  Port=3
  CoolMflw : Inport  Port=4
  JacArea : Inport  Port=5
  Divide2 : Product  Inputs=*/
  Gain4 : Gain  Gain=0.5
  LPF with IC1 : Subsystem  mask{wc=10, InitCond=EnvAirTemp, dataType=off}
      mask prompts: wc "Cutoff frequency, wc [rad/s]"; InitCond "Initial condition, InitCond [same as u]"; dataType "Enforce same input data type"
  Minus3 : Sum
  Minus4 : Sum
  Product1 : Product  Inputs=3
  Product2 : Product
  Selector : Selector  InputPortWidth=PlntEMNum  IndexOptions=Index vector (dialog)  Indices=1  OutputSizes=1
  Specific Heat 2 : Lookup_n-D  NumberOfTableDimensions=1  BreakpointsForDimension1=PlntThrCoolCpBpt  Table=PlntThrCoolCp  ExtrapMethod=Clip  UseLastTableValue=on  InternalRulePriority=Speed  RndMeth=Simplest
  Subtract : Sum  Inputs=+-
  div0protect - abs poly4 : autolibutils/div0protect - abs poly  thresh=.001  aMode=1
  BulkCoolTemp : Outport
  Qem : Outport  Port=2
  CoolTempOut : Outport  Port=3
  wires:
  LPF with IC1/1(y) -> BulkCoolTemp/1, [BulkCoolTemp]
  EMTemp/1 -> Selector/1
  HTC/1 -> Product1/1
  Product2/1 -> div0protect - abs poly4/1
  Minus4/1 -> Gain4/1
  Gain4/1 -> LPF with IC1/1(u)
  Minus3/1 -> Minus4/2, CoolTempOut/1
  Product1/1 -> Divide2/1, Qem/1  "Qem"
  JacArea/1 -> Product1/2
  div0protect - abs poly4/1 -> Divide2/2
  Specific Heat 2/1 -> Product2/2
  [BulkCoolTemp] -> Specific Heat 2/1, Subtract/2
  Subtract/1 -> Product1/3
  Selector/1 -> Subtract/1
  Divide2/1 -> Minus3/2
  CoolMflw/1 -> Product2/1
  CoolTempIn/1 -> Minus4/1, Minus3/1

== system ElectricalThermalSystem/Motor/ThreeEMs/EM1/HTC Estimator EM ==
  FluidTemp : Inport
  MassFlow : Inport  Port=2
  CrossA : Inport  Port=3  OutMin=eps
  HydDia : Inport  Port=4
  TubLen : Inport  Port=5
  Abs Viscosity : Lookup_n-D  NumberOfTableDimensions=1  BreakpointsForDimension1=PlntThrCoolCpBpt  Table=PlntThrCoolVisc  ExtrapMethod=Clip  UseLastTableValue=on  InternalRulePriority=Speed  RndMeth=Simplest
  Calculation1 : Fcn  Expr=u(1)^0.8*u(2)^0.33
  Calculation2 : Fcn  Expr=0.036*u(1)*u(2)^0.055
  Divide : Product  Inputs=**//
  Divide2 : Product  Inputs=*/
  Divide3 : Product  Inputs=*/
  Gain : Gain  Gain=0.023
  Math Function : Math  Operator=reciprocal
  Prandtl Number : Lookup_n-D  NumberOfTableDimensions=1  BreakpointsForDimension1=PlntThrCoolCpBpt  Table=PlntThrCoolPrand  ExtrapMethod=Clip  UseLastTableValue=on  InternalRulePriority=Speed  RndMeth=Simplest
  Product1 : Product
  Switch5 : Switch  Threshold=400
  Thermal Conductivity : Lookup_n-D  NumberOfTableDimensions=1  BreakpointsForDimension1=PlntThrCoolCpBpt  Table=PlntThrCoolCond  ExtrapMethod=Clip  UseLastTableValue=on  InternalRulePriority=Speed  RndMeth=Simplest
  Transfer Fcn1 : TransferFcn  Denominator=[0.1 1]
  Vector Concatenate : Concatenate
  Vector Concatenate1 : Concatenate
  HTC : Outport
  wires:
  Transfer Fcn1/1 -> HTC/1  "HTCest"
  FluidTemp/1 -> Prandtl Number/1, [CoolTemp], Abs Viscosity/1
  [CoolTemp] -> Thermal Conductivity/1
  MassFlow/1 -> Divide/1
  HydDia/1 -> [HydD], Divide/2
  CrossA/1 -> Divide/3
  [HydD] -> Divide2/1
  TubLen/1 -> Divide2/2
  Divide2/1 -> [DoL]
  Abs Viscosity/1 -> Divide/4
  Divide/1 -> Vector Concatenate1/1  "ReD"
  Prandtl Number/1 -> Vector Concatenate1/2
  Vector Concatenate1/1 -> Calculation1/1
  [DoL] -> Math Function/1
  Math Function/1 -> Switch5/2
  Thermal Conductivity/1 -> Divide3/1
  [HydD] -> Divide3/2
  Divide3/1 -> Product1/1
  Gain/1 -> Switch5/1
  Calculation1/1 -> [RePr], Gain/1
  [RePr] -> Vector Concatenate/1
  [DoL] -> Vector Concatenate/2
  Vector Concatenate/1 -> Calculation2/1
  Calculation2/1 -> Switch5/3
  Switch5/1 -> Product1/2  "NuD"
  Product1/1 -> Transfer Fcn1/1

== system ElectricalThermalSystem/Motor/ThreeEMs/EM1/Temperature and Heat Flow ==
  HTC : Inport
  CoolTempIn : Inport  Port=2
  EMTemp : Inport  Port=3
  CoolMflw : Inport  Port=4
  JacArea : Inport  Port=5
  Divide2 : Product  Inputs=*/
  Gain4 : Gain  Gain=0.5
  LPF with IC1 : Subsystem  mask{wc=10, InitCond=EnvAirTemp, dataType=off}
      mask prompts: wc "Cutoff frequency, wc [rad/s]"; InitCond "Initial condition, InitCond [same as u]"; dataType "Enforce same input data type"
  Minus3 : Sum
  Minus4 : Sum
  Product1 : Product  Inputs=3
  Product2 : Product
  Selector : Selector  InputPortWidth=PlntEMNum  IndexOptions=Index vector (dialog)  Indices=1  OutputSizes=1
  Specific Heat 2 : Lookup_n-D  NumberOfTableDimensions=1  BreakpointsForDimension1=PlntThrCoolCpBpt  Table=PlntThrCoolCp  ExtrapMethod=Clip  UseLastTableValue=on  InternalRulePriority=Speed  RndMeth=Simplest
  Subtract : Sum  Inputs=+-
  div0protect - abs poly4 : autolibutils/div0protect - abs poly  thresh=.001  aMode=1
  BulkCoolTemp : Outport
  Qem : Outport  Port=2
  CoolTempOut : Outport  Port=3
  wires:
  LPF with IC1/1(y) -> BulkCoolTemp/1, [BulkCoolTemp]
  EMTemp/1 -> Selector/1
  HTC/1 -> Product1/1
  Product2/1 -> div0protect - abs poly4/1
  Minus4/1 -> Gain4/1
  Gain4/1 -> LPF with IC1/1(u)
  Minus3/1 -> Minus4/2, CoolTempOut/1
  Product1/1 -> Divide2/1, Qem/1  "Qem"
  JacArea/1 -> Product1/2
  div0protect - abs poly4/1 -> Divide2/2
  Specific Heat 2/1 -> Product2/2
  [BulkCoolTemp] -> Specific Heat 2/1, Subtract/2
  Subtract/1 -> Product1/3
  Selector/1 -> Subtract/1
  Divide2/1 -> Minus3/2
  CoolMflw/1 -> Product2/1
  CoolTempIn/1 -> Minus4/1, Minus3/1

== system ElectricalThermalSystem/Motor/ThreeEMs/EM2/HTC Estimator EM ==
  FluidTemp : Inport
  MassFlow : Inport  Port=2
  CrossA : Inport  Port=3  OutMin=eps
  HydDia : Inport  Port=4
  TubLen : Inport  Port=5
  Abs Viscosity : Lookup_n-D  NumberOfTableDimensions=1  BreakpointsForDimension1=PlntThrCoolCpBpt  Table=PlntThrCoolVisc  ExtrapMethod=Clip  UseLastTableValue=on  InternalRulePriority=Speed  RndMeth=Simplest
  Calculation1 : Fcn  Expr=u(1)^0.8*u(2)^0.33
  Calculation2 : Fcn  Expr=0.036*u(1)*u(2)^0.055
  Divide : Product  Inputs=**//
  Divide2 : Product  Inputs=*/
  Divide3 : Product  Inputs=*/
  Gain : Gain  Gain=0.023
  Math Function : Math  Operator=reciprocal
  Prandtl Number : Lookup_n-D  NumberOfTableDimensions=1  BreakpointsForDimension1=PlntThrCoolCpBpt  Table=PlntThrCoolPrand  ExtrapMethod=Clip  UseLastTableValue=on  InternalRulePriority=Speed  RndMeth=Simplest
  Product1 : Product
  Switch5 : Switch  Threshold=400
  Thermal Conductivity : Lookup_n-D  NumberOfTableDimensions=1  BreakpointsForDimension1=PlntThrCoolCpBpt  Table=PlntThrCoolCond  ExtrapMethod=Clip  UseLastTableValue=on  InternalRulePriority=Speed  RndMeth=Simplest
  Transfer Fcn1 : TransferFcn  Denominator=[0.1 1]
  Vector Concatenate : Concatenate
  Vector Concatenate1 : Concatenate
  HTC : Outport
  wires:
  Transfer Fcn1/1 -> HTC/1  "HTCest"
  FluidTemp/1 -> Prandtl Number/1, [CoolTemp], Abs Viscosity/1
  [CoolTemp] -> Thermal Conductivity/1
  MassFlow/1 -> Divide/1
  HydDia/1 -> [HydD], Divide/2
  CrossA/1 -> Divide/3
  [HydD] -> Divide2/1
  TubLen/1 -> Divide2/2
  Divide2/1 -> [DoL]
  Abs Viscosity/1 -> Divide/4
  Divide/1 -> Vector Concatenate1/1  "ReD"
  Prandtl Number/1 -> Vector Concatenate1/2
  Vector Concatenate1/1 -> Calculation1/1
  [DoL] -> Math Function/1
  Math Function/1 -> Switch5/2
  Thermal Conductivity/1 -> Divide3/1
  [HydD] -> Divide3/2
  Divide3/1 -> Product1/1
  Gain/1 -> Switch5/1
  Calculation1/1 -> [RePr], Gain/1
  [RePr] -> Vector Concatenate/1
  [DoL] -> Vector Concatenate/2
  Vector Concatenate/1 -> Calculation2/1
  Calculation2/1 -> Switch5/3
  Switch5/1 -> Product1/2  "NuD"
  Product1/1 -> Transfer Fcn1/1

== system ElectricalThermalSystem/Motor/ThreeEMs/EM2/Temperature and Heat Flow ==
  HTC : Inport
  CoolTempIn : Inport  Port=2
  EMTemp : Inport  Port=3
  CoolMflw : Inport  Port=4
  JacArea : Inport  Port=5
  Divide2 : Product  Inputs=*/
  Gain4 : Gain  Gain=0.5
  LPF with IC1 : Subsystem  mask{wc=10, InitCond=EnvAirTemp, dataType=off}
      mask prompts: wc "Cutoff frequency, wc [rad/s]"; InitCond "Initial condition, InitCond [same as u]"; dataType "Enforce same input data type"
  Minus3 : Sum
  Minus4 : Sum
  Product1 : Product  Inputs=3
  Product2 : Product
  Selector : Selector  InputPortWidth=PlntEMNum  IndexOptions=Index vector (dialog)  Indices=2  OutputSizes=1
  Specific Heat 2 : Lookup_n-D  NumberOfTableDimensions=1  BreakpointsForDimension1=PlntThrCoolCpBpt  Table=PlntThrCoolCp  ExtrapMethod=Clip  UseLastTableValue=on  InternalRulePriority=Speed  RndMeth=Simplest
  Subtract : Sum  Inputs=+-
  div0protect - abs poly4 : autolibutils/div0protect - abs poly  thresh=.001  aMode=1
  BulkCoolTemp : Outport
  Qem : Outport  Port=2
  CoolTempOut : Outport  Port=3
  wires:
  LPF with IC1/1(y) -> BulkCoolTemp/1, [BulkCoolTemp]
  EMTemp/1 -> Selector/1
  HTC/1 -> Product1/1
  Product2/1 -> div0protect - abs poly4/1
  Minus4/1 -> Gain4/1
  Gain4/1 -> LPF with IC1/1(u)
  Minus3/1 -> Minus4/2, CoolTempOut/1
  Product1/1 -> Divide2/1, Qem/1  "Qem"
  JacArea/1 -> Product1/2
  div0protect - abs poly4/1 -> Divide2/2
  Specific Heat 2/1 -> Product2/2
  [BulkCoolTemp] -> Specific Heat 2/1, Subtract/2
  Subtract/1 -> Product1/3
  Selector/1 -> Subtract/1
  Divide2/1 -> Minus3/2
  CoolMflw/1 -> Product2/1
  CoolTempIn/1 -> Minus4/1, Minus3/1
